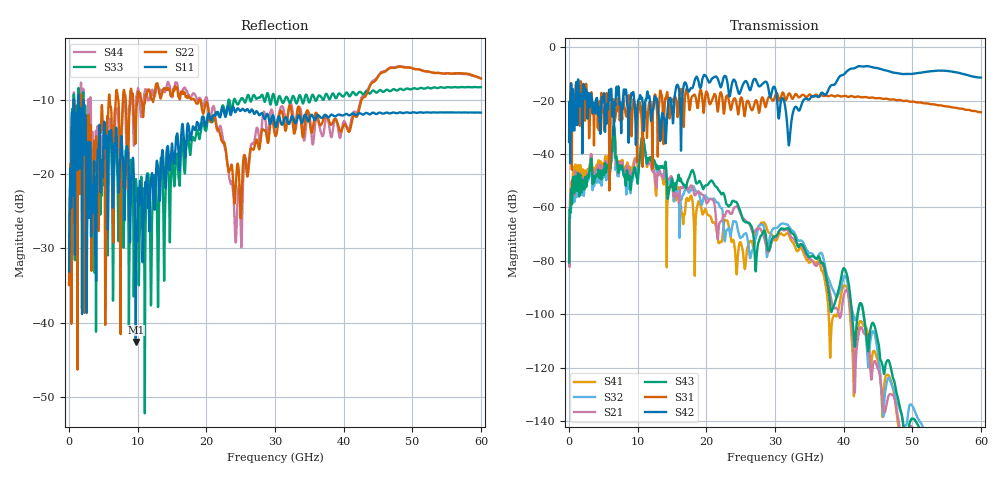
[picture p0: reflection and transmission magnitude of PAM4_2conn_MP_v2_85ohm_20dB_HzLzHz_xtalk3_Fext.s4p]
! Info: Touchstone file created by Circ.  Input file=FAB50GbE_2conn_Midplane_Examax_Topo2_v2_85ohm_20dB_HzLzHz.circ
# Hz S RI R 50
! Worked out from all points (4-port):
!   6000 points, 10 MHz to 60 GHz, reference 50 ohm
!   strongest paths, dB at 10 MHz, 15.01 GHz, 30.01 GHz, 45.01 GHz, 60 GHz:
!     S42: -35.5, -24.0, -15.3, -7.9, -11.4
!     S31: -35.3, -19.6, -18.3, -19.1, -24.4
!     S43: -80.6, -49.3, -71.0, -109.9, -160.5
!     S21: -64.0, -49.5, -71.6, -120.4, -158.4
!     S32: -68.1, -48.8, -67.8, -114.7, -152.9
!     S41: -67.5, -51.2, -72.3, -117.6, -169.5
!   lowest |S11| = -42.6 dB at 9.72 GHz (marker M1), VSWR 1.01, Z = 50.7 + j0.29 ohm
!   |S11| at or under -10 dB: start of sweep to 682.6 MHz; 714.8 MHz to 1.334 GHz (619 MHz wide, 60.4 % of centre); 1.444 GHz to end of sweep
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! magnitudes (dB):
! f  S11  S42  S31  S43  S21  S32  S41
! 10 MHz  -33.1  -35.5  -35.3  -80.6  -64.0  -68.1  -67.5
! 780 MHz  -13.5  -29.6  -20.9  -54.3  -54.7  -58.0  -51.0
! 6.44 GHz  -23.6  -22.9  -19.6  -30.6  -32.8  -34.3  -31.1
! 9.72 GHz  -42.6  -34.9  -25.0  -47.0  -41.9  -45.4  -41.8
! 24.41 GHz  -11.3  -14.5  -21.3  -58.1  -59.6  -66.0  -85.1
! 32.06 GHz  -13.2  -36.5  -17.3  -68.1  -69.6  -67.2  -70.6
! 60 GHz  -11.7  -11.4  -24.4  -160.5  -158.4  -152.9  -169.5
